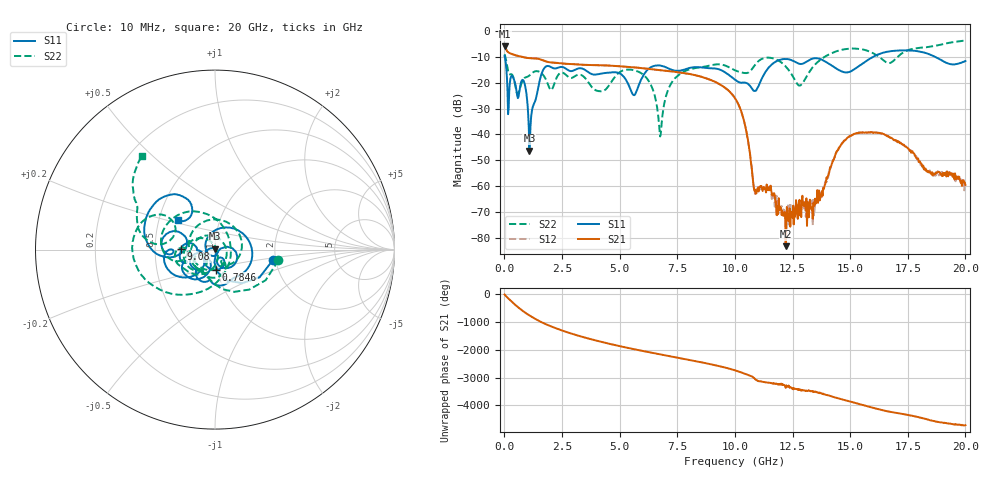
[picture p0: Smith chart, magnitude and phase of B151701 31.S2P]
!  2-Port S-parameters saved by WinCal
! VAR MeasName=S-Parameters (CALIBRATED_DATA) read from VNA (N5244A)
! VAR MeasDate=2015-12-24 19:12:52
! VAR NAME=B151701 31
! VAR FILENAME=B151701 31.S2P
! VAR DATE=2015-12-24 19:12:52
! VAR PHYS_PORTS=1,3
# Hz S DB R 50
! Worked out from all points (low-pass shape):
!   801 points, 10 MHz to 20 GHz, reference 50 ohm
!   highest |S21| = -5.91 dB at 10 MHz (marker M1); lowest = -83.3 dB at 12.2 GHz (marker M2)
!   |S21| within 3 dB of the highest: start of sweep to 343.6 MHz
!   lowest |S11| = -46.3 dB at 1.084 GHz (marker M3), VSWR 1.01, Z = 50 + j0.482 ohm
!   |S11| at or under -10 dB: 18.53 MHz to 15.98 GHz (15.96 GHz wide, 200 % of centre); 18.7 GHz to end of sweep
!   |S22| runs from -40.8 to -3.6 dB; largest |S21 - S12| = 0.001
!   S11 on the Smith chart (normalised r, x): 10 MHz: 1.94, -0.24; 784.6 MHz: 0.99, -0.23; 9.08 GHz: 0.68, +0.00; 20 GHz: 0.63, +0.22
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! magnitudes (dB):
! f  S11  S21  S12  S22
! 10 MHz  -9.6  -5.9  -5.9  -8.9
! 209.9 MHz  -23.4  -8.4  -8.4  -16.7
! 784.6 MHz  -18.8  -10.0  -10.0  -19.2
! 1.084 GHz  -46.3  -10.4  -10.4  -17.2
! 1.759 GHz  -14.0  -11.6  -11.6  -18.0
! 3.358 GHz  -14.4  -13.0  -13.0  -17.1
! 4.183 GHz  -16.5  -13.2  -13.2  -23.3
! 5.607 GHz  -24.7  -14.0  -14.0  -15.1
! 5.907 GHz  -19.2  -14.3  -14.3  -16.1
! 6.407 GHz  -13.7  -14.8  -14.8  -21.8
! 6.682 GHz  -13.3  -15.1  -15.1  -33.5
! 7.456 GHz  -15.3  -15.8  -15.8  -17.8
! 9.08 GHz  -14.4  -19.4  -19.4  -13.0
! 10.01 GHz  -18.8  -26.0  -26.0  -15.2
! 10.45 GHz  -19.9  -37.0  -37.0  -16.2
! 10.88 GHz  -23.2  -61.4  -63.2  -13.0
! 12.2 GHz  -10.7  -83.3  -72.1  -13.7
! 12.8 GHz  -12.6  -65.4  -65.4  -21.1
! 13.35 GHz  -10.7  -68.3  -65.6  -14.2
! 14.78 GHz  -15.9  -42.3  -42.2  -7.0
! 16.68 GHz  -7.8  -40.9  -40.9  -12.4
! 20 GHz  -11.6  -59.6  -59.6  -3.6
